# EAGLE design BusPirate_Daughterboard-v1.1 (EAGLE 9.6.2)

## Sheet 1 of 2: Power
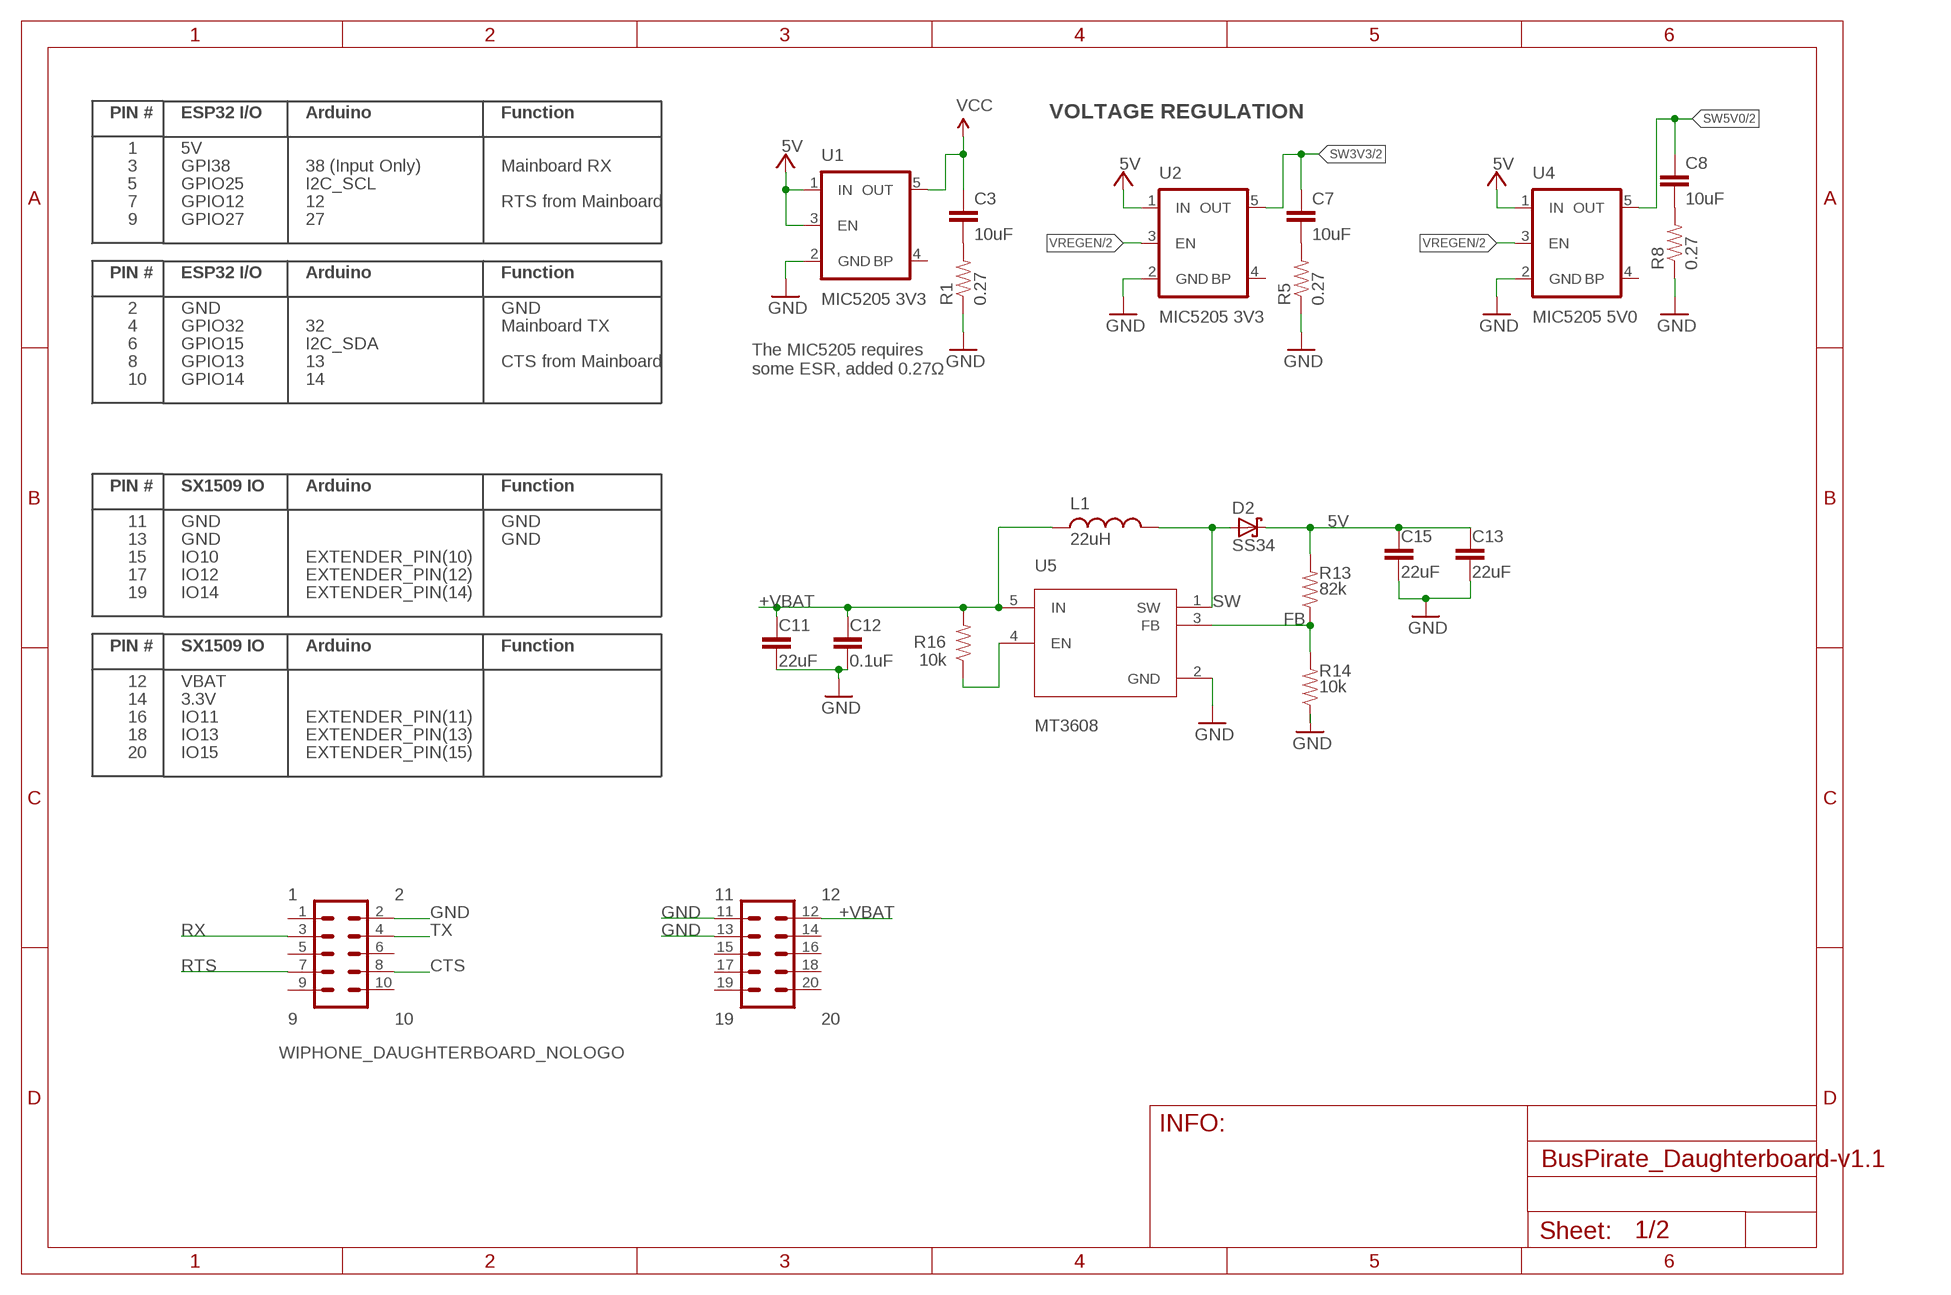
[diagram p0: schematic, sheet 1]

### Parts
C3  10uF  CAP0805  [0805_CAP]
C7  10uF  CAP0805  [0805_CAP]
C8  10uF  CAP0805  [0805_CAP]
C11  22uF  CAP0805  [0805_CAP]
C12  0.1uF  CAP0603  [0603-CAP]
C13  22uF  CAP0805  [0805_CAP]
C15  22uF  CAP0805  [0805_CAP]
D2  SS34  DIODE_SCHOTTKEY  [SOD323]
JP3  WIPHONE_DAUGHTERBOARD_NOLOGO  [WIPHONE_DAUGHTERBOARD-NL]
L1  22uH  IND0420  [0420-IND]
R1  0.27  RES0603  [0603-RES]
R5  0.27  RES0603  [0603-RES]
R8  0.27  RES0603  [0603-RES]
R13  82k  RES0603  [0603-RES]
R14  10k  RES0603  [0603-RES]
R16  10k  RES0603  [0603-RES]
U1  MIC5205 3V3  MIC5205-3.3V  [SOT23-5(SOT95P280X130-5-M)]
U2  MIC5205 3V3  MIC5205-3.3V  [SOT23-5(SOT95P280X130-5-M)]
U4  MIC5205 5V0  MIC5205-5V  [SOT23-5(SOT95P280X130-5-M)]
U5  MT3608  [SOT95P280X145-6N]

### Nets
5V: C13.2 C15.2 D2.C R13.2 U1.1(IN) U1.3(EN) U2.1(IN) U4.1(IN) ; also sheet 2
+VBAT: C11.2 C12.2 JP3.12 L1.1 R16.2 U5.5(IN)
CTS: JP3.8 ; also sheet 2
FB: R13.1 R14.2 U5.3(FB)
GND: C11.1 C12.1 C13.1 C15.1 JP3.2 JP3.11 JP3.13 R1.1 R5.1 R8.1 R14.1 U1.2(GND) U2.2(GND) U4.2(GND) U5.2(GND) ; also sheet 2
N$8: C3.2 R1.2
N$10: C7.2 R5.2
N$11: C8.2 R8.2
N$12: R16.1 U5.4(EN)
RTS: JP3.7 ; also sheet 2
RX: JP3.3 ; also sheet 2
SW: D2.A L1.2 U5.1(SW)
SW3V3: C7.1 U2.5(OUT) ; also sheet 2
SW5V0: C8.1 U4.5(OUT) ; also sheet 2
TX: JP3.4 ; also sheet 2
VCC: C3.1 U1.5(OUT) ; also sheet 2
VREGEN: U2.3(EN) U4.3(EN) ; also sheet 2
Unconnected: JP3.5 JP3.6 JP3.9 JP3.10 JP3.15 JP3.16 JP3.17 JP3.18 JP3.19 JP3.20 U1.4(BP) U2.4(BP) U4.4(BP)

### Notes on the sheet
- VOLTAGE REGULATION
- Mainboard RX
- RTS from Mainboard
- GND
- Mainboard TX
- CTS from Mainboard
- The MIC5205 requires
  some ESR, added 0.27Ω
- GND
- GND

## Sheet 2 of 2: Microcontroller
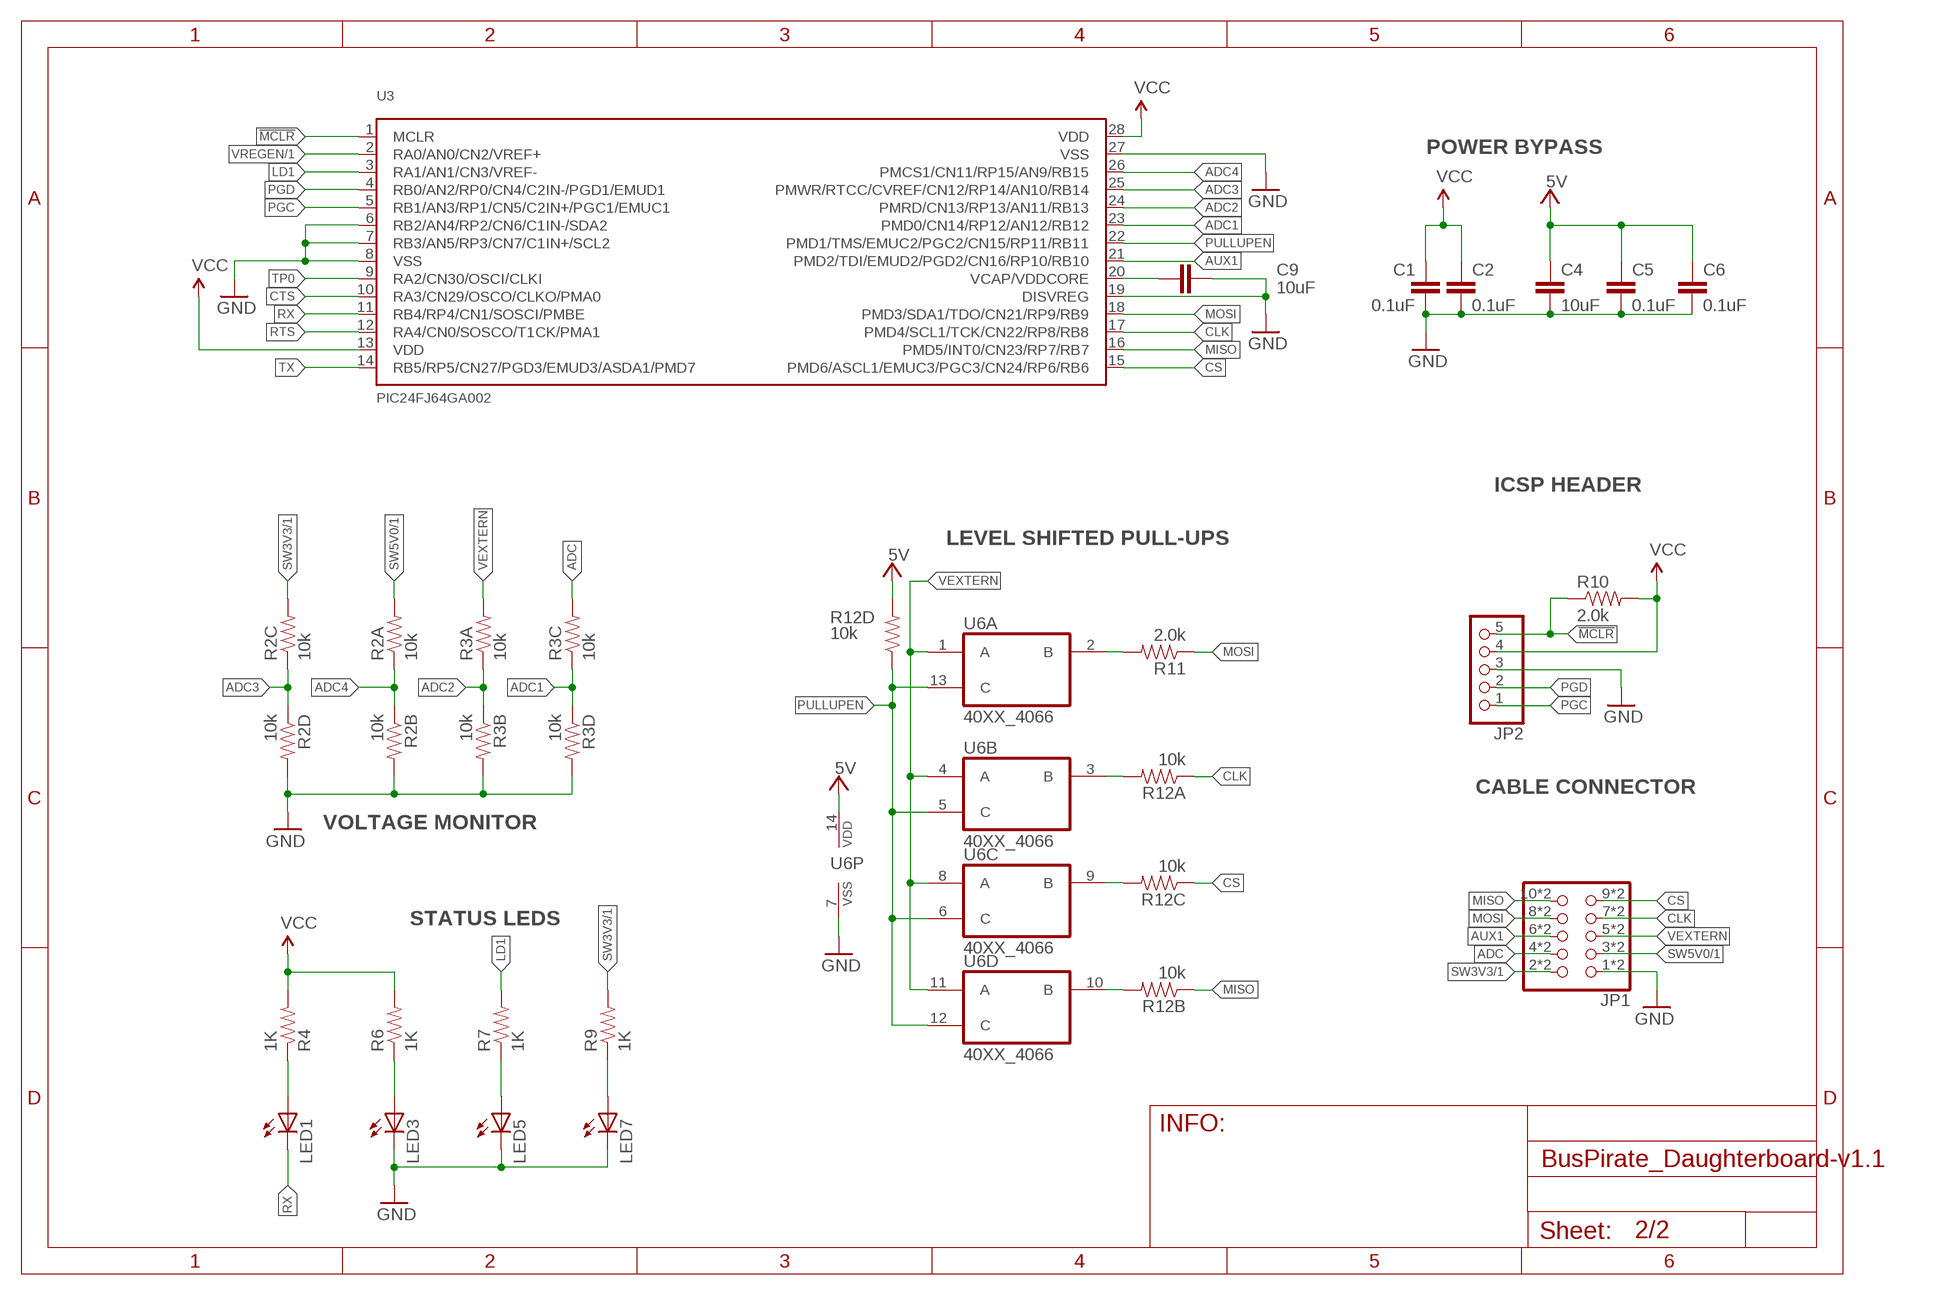
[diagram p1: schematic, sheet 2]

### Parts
C1  0.1uF  CAP0603  [0603-CAP]
C2  0.1uF  CAP0603  [0603-CAP]
C4  10uF  CAP0805  [0805_CAP]
C5  0.1uF  CAP0603  [0603-CAP]
C6  0.1uF  CAP0603  [0603-CAP]
C9  10uF  CAP0805  [0805_CAP]
JP1  PINHD-2X5-M05X2SHD_SMD  [M05X2SHD_SMD]
JP2  PINHD-1X5  [1X05]
LED1  RED  LED0603  [0603-LED]
LED3  RED  LED0603  [0603-LED]
LED5  RED  LED0603  [0603-LED]
LED7  RED  LED0603  [0603-LED]
R2  10k  RES_CAY16-F4  [RES_4XARRAY]
R3  10k  RES_CAY16-F4  [RES_4XARRAY]
R4  1K  RES0603  [0603-RES]
R6  1K  RES0603  [0603-RES]
R7  1K  RES0603  [0603-RES]
R9  1K  RES0603  [0603-RES]
R10  2.0k  RES0603  [0603-RES]
R11  2.0k  RES0603  [0603-RES]
R12  10k  RES_CAY16-F4  [RES_4XARRAY]
U3  PIC24FJ64GA002  [SSOP-28(SSOP65P780X200-28-M)]
U6  40XX_4066  [TSSOP-14(SOP65P660X120-14-M)]

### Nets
5V: C4.1 C5.1 C6.1 R12.5 U6.14(P:VDD) ; also sheet 1
!MCLR: JP2.5 R10.1 U3.1(MCLR)
ADC: JP1.4 JP1.14 R3.6
ADC1: R3.3 R3.4 U3.23(PMD0/CN14/RP12/AN12/RB12)
ADC2: R3.1 R3.2 U3.24(PMRD/CN13/RP13/AN11/RB13)
ADC3: R2.3 R2.4 U3.25(PMWR/RTCC/CVREF/CN12/RP14/AN10/RB14)
ADC4: R2.1 R2.2 U3.26(PMCS1/CN11/RP15/AN9/RB15)
AUX1: JP1.6 JP1.16 U3.21(PMD2/TDI/EMUD2/PGD2/CN16/RP10/RB10)
CLK: JP1.7 JP1.17 R12.1 U3.17(PMD4/SCL1/TCK/CN22/RP8/RB8)
CS: JP1.9 JP1.19 R12.3 U3.15(PMD6/ASCL1/EMUC3/PGC3/CN24/RP6/RB6)
CTS: U3.10(RA3/CN29/OSCO/CLKO/PMA0) ; also sheet 1
GND: C1.2 C2.2 C4.2 C5.2 C6.2 C9.2 JP1.1 JP1.11 JP2.3 LED3.C LED5.C LED7.C R2.5 R2.7 R3.5 R3.7 U3.6(RB2/AN4/RP2/CN6/C1IN-/SDA2) U3.7(RB3/AN5/RP3/CN7/C1IN+/SCL2) U3.8(VSS) U3.19(DISVREG) U3.27(VSS) U6.7(P:VSS) ; also sheet 1
LD1: R7.2 U3.3(RA1/AN1/CN3/VREF-)
MISO: JP1.10 JP1.20 R12.2 U3.16(PMD5/INT0/CN23/RP7/RB7)
MOSI: JP1.8 JP1.18 R11.1 U3.18(PMD3/SDA1/TDO/CN21/RP9/RB9)
N$1: R11.2 U6.2(A:B)
N$2: R12.6 U6.9(C:B)
N$3: C9.1 U3.20(VCAP/VDDCORE)
N$4: R12.7 U6.10(D:B)
N$5: R12.8 U6.3(B:B)
N$6: LED5.A R7.1
N$7: LED3.A R6.1
N$13: LED1.A R4.1
N$18: LED7.A R9.1
PGC: JP2.1 U3.5(RB1/AN3/RP1/CN5/C2IN+/PGC1/EMUC1)
PGD: JP2.2 U3.4(RB0/AN2/RP0/CN4/C2IN-/PGD1/EMUD1)
PULLUPEN: R12.4 U3.22(PMD1/TMS/EMUC2/PGC2/CN15/RP11/RB11) U6.5(B:C) U6.6(C:C) U6.12(D:C) U6.13(A:C)
RTS: U3.12(RA4/CN0/SOSCO/T1CK/PMA1) ; also sheet 1
RX: LED1.C U3.11(RB4/RP4/CN1/SOSCI/PMBE) ; also sheet 1
SW3V3: JP1.2 JP1.12 R2.6 R9.2 ; also sheet 1
SW5V0: JP1.3 JP1.13 R2.8 ; also sheet 1
TP0: U3.9(RA2/CN30/OSCI/CLKI)
TX: U3.14(RB5/RP5/CN27/PGD3/EMUD3/ASDA1/PMD7) ; also sheet 1
VCC: C1.1 C2.1 JP2.4 R4.2 R6.2 R10.2 U3.13(VDD) U3.28(VDD) ; also sheet 1
VEXTERN: JP1.5 JP1.15 R3.8 U6.1(A:A) U6.4(B:A) U6.8(C:A) U6.11(D:A)
VREGEN: U3.2(RA0/AN0/CN2/VREF+) ; also sheet 1

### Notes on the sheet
- POWER BYPASS
- ICSP HEADER
- LEVEL SHIFTED PULL-UPS
- CABLE CONNECTOR
- VOLTAGE MONITOR
- STATUS LEDS

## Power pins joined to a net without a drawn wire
1: JP3.1
14: JP3.14

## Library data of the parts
C1-C9 C11-C13 C15 = HackEDA V1.0:CAP: Capacitor.
D2 = HackEDA V1.0:DIODE_SCHOTTKEY: Schottky barrier diode
JP1 = HackEDA V1.0:PINHD-2X5: PIN HEADER; PROD_ID: CONN-09508
JP2 = HackEDA V1.0:PINHD-1X5: PIN HEADER
JP3 = WiPhone:WIPHONE_DAUGHTERBOARD
L1 = HackEDA V1.0:IND: Inductor.
LED1 LED3 LED5 LED7 = HackEDA V1.0:LED: LED.
R1 R4-R11 R13 R14 R16 = HackEDA V1.0:RES: Resistor.
R2 R3 R12 = HackEDA V1.0:RES_CAY16-F4: CAY16-F4; PROD_ID: RES-13167
U1 U2 U4 = HackEDA V1.0:MIC5205: MIC5205 150mA vreg 3.3V - VREG-00822 5V - VREG-00823
U3 = HackEDA V1.0:PIC24FJ64GA002: 16-bit General Purpose Flash Microcontroller
U5 = HackEDA V1.0:MT3608: High Efficiency 1.2MHz 2A Step Up Converter; DESCRIPTION: High Efficiency 1.2MHz 2A Step Up Converter; MF: Aerosemi Technology Co., Ltd; MP: MT3608; PACKAGE: Package
U6 = HackEDA V1.0:40XX_4066: Quad bilateral ANALOG SWITCH; PROD_ID: IC-13191

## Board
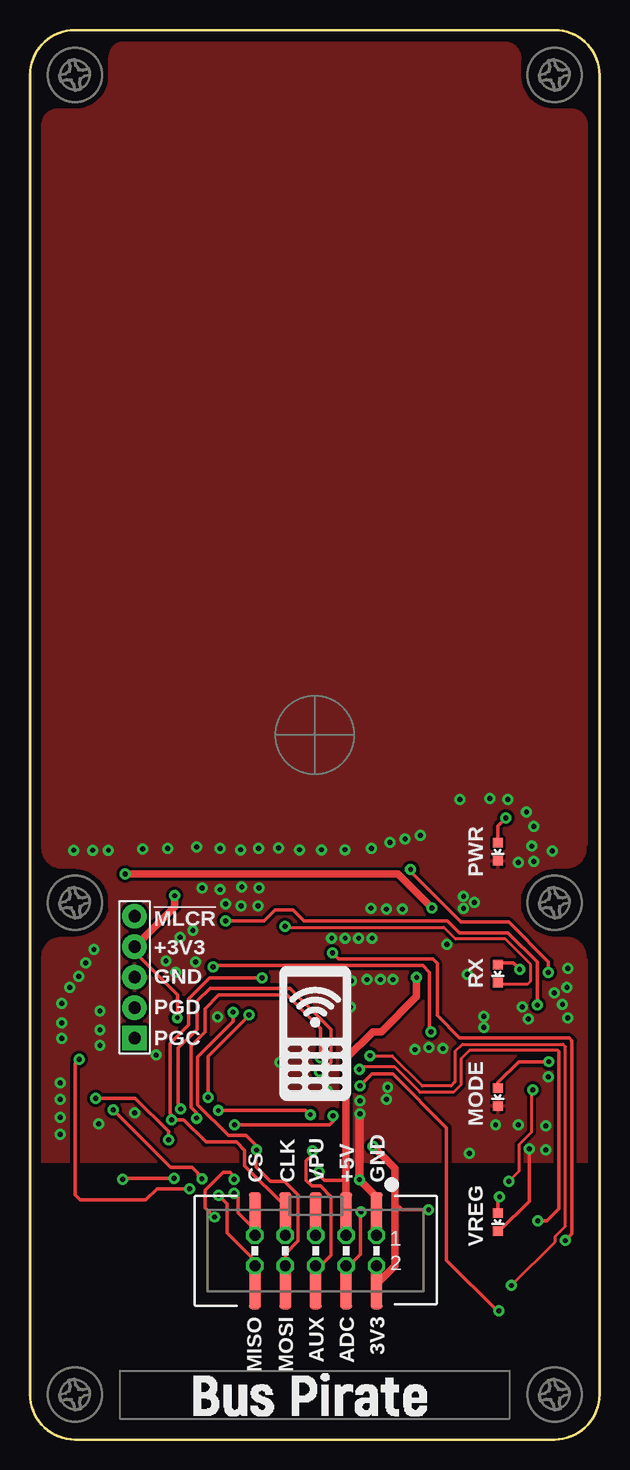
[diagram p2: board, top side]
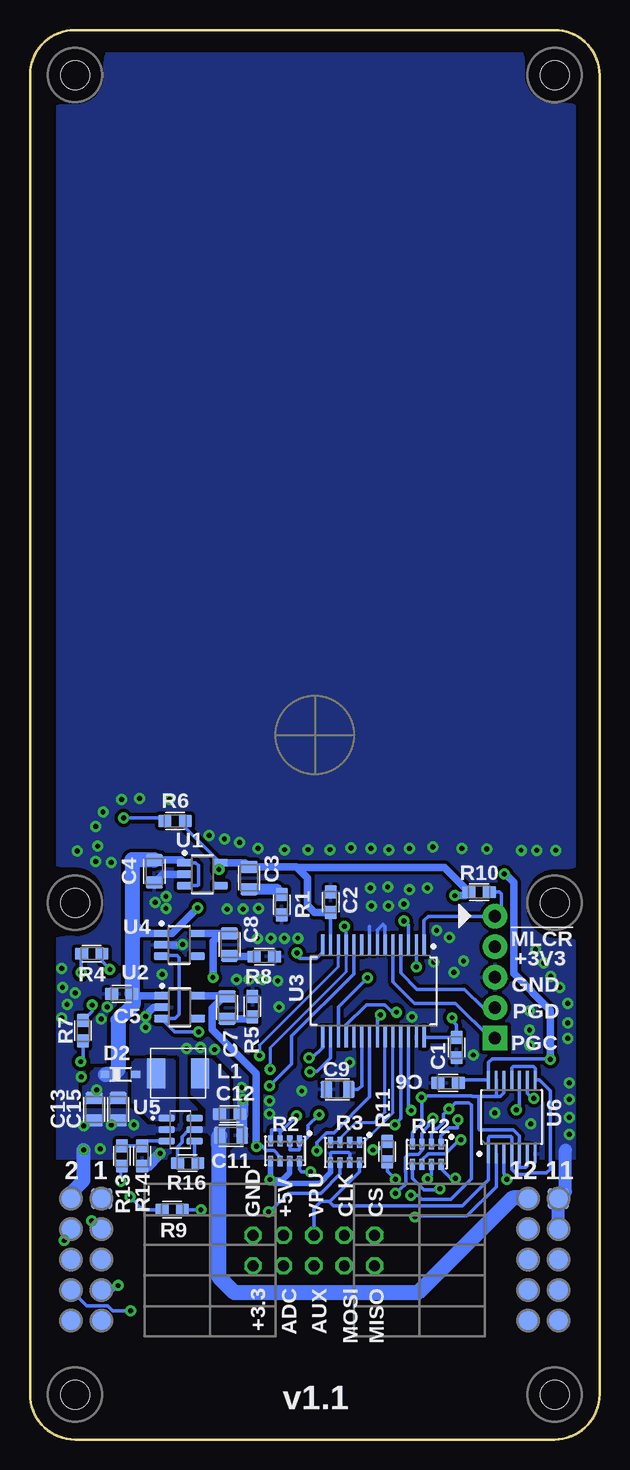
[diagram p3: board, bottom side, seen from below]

Size 47.5 x 117.5 mm. Coordinates in mm from the lower left corner, seen from the top.
Copper layers (1*16): Top 0.035mm / dielectric 1.5mm / Bottom 0.035mm
Design rules "MZJ_2Layer_Standard *": minimum track width 10mil, minimum drill 16mil, track to track 10mil, track to pad 8mil, pad to pad 8mil, via to via 10mil, smd to smd 0mil, copper to edge 8mil, drill to drill 8mil, minimum pad ring 10mil, minimum via ring 10mil, stop-mask expansion 4mil, vias tented up to drill 25mil, thermal gap 10mil
bRestrict: area 18.1,40.5 to 18.3,42.1; area 18.7,40.4 to 19,42; area 19.4,40.4 to 19.6,42; area 6.2,23 to 6.4,24.6

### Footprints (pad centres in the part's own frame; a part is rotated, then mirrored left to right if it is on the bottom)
0603-CAP = smd 1.1 x 1: 1 -0.85,0; 2 0.85,0
0805_CAP = smd 1 x 1.42: 1 -0.935,0; 2 0.935,0
SOD323 = smd 0.8 x 0.6: A 1.25,0; C -1.25,0
M05X2SHD_SMD = smd 4.15 x 1: 1 -2.794,5.08; 2 2.794,5.08; 3 -2.794,2.54; 4 2.794,2.54; 5 -2.794,0; 6 2.794,0; 7 -2.794,-2.54; 8 2.794,-2.54; 9 -2.794,-5.08; 10 2.794,-5.08 | drill 0.914 octagon: 11 -1.27,5.08; 12 1.27,5.08; 13 -1.27,2.54; 14 1.27,2.54; 15 -1.27,0; 16 1.27,0; 17 -1.27,-2.54; 18 1.27,-2.54; 19 -1.27,-5.08; 20 1.27,-5.08
1X05 = drill 1.016 pad 2.032 square: 1 -5.08,0 | drill 1.016 pad 2.032: 2 -2.54,0; 3 0,0; 4 2.54,0; 5 5.08,0
WIPHONE_DAUGHTERBOARD-NL = smd 1.75 x 1.75 bottom: 1 17.78,-38.66; 2 20.32,-38.66; 3 17.78,-41.2; 4 20.32,-41.2; 5 17.78,-43.74; 6 20.32,-43.74; 7 17.78,-46.28; 8 20.32,-46.28; 9 17.78,-48.82; 10 20.32,-48.82; 11 -20.32,-38.66; 12 -17.78,-38.66; 13 -20.32,-41.2; 14 -17.78,-41.2; 15 -20.32,-43.74; 16 -17.78,-43.74; 17 -20.32,-46.28; 18 -17.78,-46.28; 19 -20.32,-48.82; 20 -17.78,-48.82 | hole 2.4: 20,-54.991; -20,-54.991; 20,-13.991; 20,55.009; -20,55.009; -20,-13.991
0420-IND = smd 1.5 x 2.5: 1 -1.85,0; 2 1.85,0
0603-LED = smd 0.8 x 0.8: A 0,-0.75; C 0,0.75
0603-RES = smd 1.1 x 1: 1 -0.85,0; 2 0.85,0
RES_4XARRAY = smd 0.425 x 0.9: 1 -1.2,-0.85; 2 -0.4,-0.85; 3 0.4,-0.85; 4 1.2,-0.85; 5 1.2,0.85; 6 0.4,0.85; 7 -0.4,0.85; 8 -1.2,0.85
SOT23-5(SOT95P280X130-5-M) = smd 1.2 x 0.6: 1 -1.528,0.95; 2 -1.528,0; 3 -1.528,-0.95; 4 1.528,-0.95; 5 1.528,0.95
SSOP-28(SSOP65P780X200-28-M) = smd 1.748 x 0.35: 1 -3.853,4.225; 2 -3.853,3.575; 3 -3.853,2.925; 4 -3.853,2.275; 5 -3.853,1.625; 6 -3.853,0.975; 7 -3.853,0.325; 8 -3.853,-0.325; 9 -3.853,-0.975; 10 -3.853,-1.625; 11 -3.853,-2.275; 12 -3.853,-2.925; 13 -3.853,-3.575; 14 -3.853,-4.225; 15 3.853,-4.225; 16 3.853,-3.575; 17 3.853,-2.925; 18 3.853,-2.275; 19 3.853,-1.625; 20 3.853,-0.975; 21 3.853,-0.325; 22 3.853,0.325; 23 3.853,0.975; 24 3.853,1.625; 25 3.853,2.275; 26 3.853,2.925; 27 3.853,3.575; 28 3.853,4.225
SOT95P280X145-6N = smd 1.37 x 0.59: 1 -1.17,0.95; 2 -1.17,0; 3 -1.17,-0.95; 4 1.17,-0.95; 5 1.17,0; 6 1.17,0.95
TSSOP-14(SOP65P660X120-14-M) = smd 1.562 x 0.32: 1 -3.075,1.95; 2 -3.075,1.3; 3 -3.075,0.65; 4 -3.075,0; 5 -3.075,-0.65; 6 -3.075,-1.3; 7 -3.075,-1.95; 8 3.075,-1.95; 9 3.075,-1.3; 10 3.075,-0.65; 11 3.075,0; 12 3.075,0.65; 13 3.075,1.3; 14 3.075,1.95

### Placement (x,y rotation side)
C1  11.93,32.68 270 bottom
C2  22.42,44.79 90 bottom
C3  29.23,46.8 270 bottom
C4  37.13,47.37 270 bottom
C5  39.85,37.15 180 bottom
C6  12.62,29.73 180 bottom
C7  31.06,36.02 270 bottom
C8  30.86,41.26 270 bottom
C9  21.85,29.18 180 bottom
C11  30.75,25.34 180 bottom
C12  30.85,27.14 180 bottom
C13  42.15,27.54 90 bottom
C15  40.15,27.54 90 bottom
D2  39.95,30.44 0 bottom
JP1  23.83,15.74 270 top
JP2  8.72,38.54 90 top
JP3  23.75,58.74 0 top
L1  35.15,30.54 180 bottom
LED1  39.02,38.84 180 top
LED3  39.02,49 180 top
LED5  39.02,28.55 180 top
LED7  39.02,18.13 180 top
R1  26.51,44.59 90 bottom
R2  26.23,24.06 180 bottom
R3  21.23,23.93 180 bottom
R4  42.35,40.51 180 bottom
R5  28.94,36.09 270 bottom
R6  35.4,51.56 0 bottom
R7  43.07,34.08 90 bottom
R8  27.95,40.27 180 bottom
R9  35.64,19.16 0 bottom
R10  10.05,45.64 180 bottom
R11  17.71,24 270 bottom
R12  14.41,23.78 180 bottom
R13  39.85,23.64 270 bottom
R14  38.15,23.64 90 bottom
R16  34.35,23.04 180 bottom
U1  33.12,47.12 0 bottom
U2  35.02,36.04 0 bottom
U3  18.85,37.39 270 bottom
U4  35.04,41.24 0 bottom
U5  34.95,25.84 0 bottom
U6  7.32,26.89 90 bottom

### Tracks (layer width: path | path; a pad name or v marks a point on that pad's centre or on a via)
5V  (via drill 0.41)
  Top 0.254: v39.95,21.54 40.8,22.38 40.8,24.59 41.85,25.64 41.85,29.14 v41.95,29.14
  Top 0.305: v13.31,20.9 10.6,20.9 9.66,19.96 4.19,19.96 3.75,20.4 3.75,31.35 v4.1,31.7
  Top 0.61: v33.52,44.33 30.71,47.14 v7.95,47.14
  Bottom 0.254: R13.2 39.95,22.69 v39.95,21.54 | v41.95,29.14 42.15,28.94 C13.2
  Bottom 0.305: C6.1 11.54,29.96 U6.14 9.26,29.98 9.26,31.42 8.94,31.74 4.09,31.74 4.05,31.7 v4.1,31.7 | v13.31,20.9 13.31,20.83 14.65,20.83 15.61,21.78 15.61,22.55 R12.5 | U1.3 33.51,46.17 33.45,46.24 33.45,47.84 33.68,48.07 U1.1
  Bottom 0.61: 38.6,42.39 38.4,42.19 U4.1 35.66,42.19 v33.52,44.33 | U2.1 38.84,36.99 C5.1 | v4.1,31.7 4.1,35.79 7.15,38.84 7.15,46.44 7.85,47.14 v7.95,47.14 | C4.1 34.88,48.3 U1.1
  Bottom 1.27: 39,42.79 39,48.32 37.15,48.32 C4.1 | 39,42.79 C5.1 38.91,37.06 38.91,36.2 40.15,34.96 40.15,30.84 40.55,30.44 D2.C | 39,42.79 38.6,42.39
  pour Bottom (rank 2, no thermals): 39.45,28.94 39.45,30.54 39.85,30.94 42.05,30.94 42.35,30.64 43.05,29.94 43.05,27.94 42.95,28.04 39.45,28.04
!MCLR
  Bottom 0.305: U3.1 14.63,43.28 14.29,43.62 8.06,43.62 | JP2.5 8.06,43.62 | R10.1 8.37,45.64 8.2,45.48 8.2,43.76 8.06,43.62
+VBAT
  Bottom 0.305: R16.2 35.2,24.41 34.82,24.79 34.82,25.24 34.22,25.84 U5.5
  Bottom 1.27: JP3.12 5.91,20.14 7.25,20.14 15.15,12.24 30.45,12.24 31.75,13.54 31.75,25.27 C11.2
  pour Bottom (no thermals): 33.55,25.64 32.75,25.64 32.35,25.24 32.35,24.54 31.05,24.54 30.95,24.64 30.95,30.24 32.35,31.64 34,31.64 34,28.79 32.75,27.54 32.75,26.14 32.85,26.04 33.55,26.04
ADC  (via drill 0.41)
  Top 0.305: JP1.14 JP1.4 26.37,14.26 27.55,15.44 27.55,18.94 v27.6,18.99
  Bottom 0.305: R3.6 21.63,22.15 23.25,20.53 25.95,20.53 27.55,18.94 v27.6,18.99
ADC1
  Bottom 0.254: R3.3 21.63,25.11 20.32,26.42 18.76,26.42 17.88,27.3 U3.23
  Bottom 0.305: R3.3 R3.4
ADC2
  Bottom 0.254: R3.1 19.69,24.78 17.23,27.23 U3.24
  Bottom 0.305: R3.2 20.83,24.71 20.01,24.71 20.01,24.76 R3.1
ADC3  (via drill 0.41)
  Top 0.305: v17.06,26.22 24.97,26.22 25.37,26.62 25.37,26.86 v25.26,26.97
  Bottom 0.305: U3.25 16.58,26.75 17.06,26.27 v17.06,26.22 | v25.26,26.97 26.52,25.72 | 26.52,25.72 26.63,25.6 R2.3 | R2.4 27.35,24.99 27.35,25.82 26.62,25.82 26.52,25.72
ADC4  (via drill 0.41)
  Top 0.305: v15.71,27.42 22.96,27.42 23.38,27 v23.38,27.08
  Bottom 0.305: U3.26 15.93,27.63 15.72,27.42 v15.71,27.42 | v23.38,27.08 24.29,26.17 24.29,25.25 24.63,24.91 R2.1 25.03,24.18 25.07,24.14 25.8,24.14 25.8,24.88 R2.2
AUX1  (via drill 0.41)
  Top 0.305: v23.58,24.05 23.57,24.04 23.57,23.75 23.04,23.21 23.04,21.6 23.5,21.13 24.23,21.13 25.12,20.24 25.12,15.34 23.83,14.05 JP1.6 JP1.16
  Bottom 0.305: U3.21 19.18,28.55 22.14,25.58 22.79,25.58 23.58,24.79 v23.58,24.05
CLK  (via drill 0.41)
  Top 0.305: JP1.17 JP1.7 21.29,19.42 17.89,22.82 17.89,24.12 17.21,24.8 14.67,24.8 12.83,26.64 v11.83,26.64 11.83,27.07 11.71,27.19 11.71,33.04 13.25,34.58 13.25,36.74 14.99,38.48 v19.36,38.48
  Bottom 0.305: v11.83,26.64 11.83,26.42 11.87,26.38 11.87,25.97 12.58,25.97 13.21,25.33 R12.1 | U3.17 21.78,36.07 v19.36,38.48
CS  (via drill 0.41)
  Top 0.305: v13.9,26.79 13.9,27.22 13.44,27.68 13.44,32.81 14.59,33.96 14.59,35.92 15.74,37.06 21.44,37.06 24.23,34.28 v24.23,31.8 | JP1.9 JP1.19 18.75,17.5 17.33,18.91 17.33,20.22 v17.03,20.52
  Bottom 0.305: U3.15 23.08,32.68 23.96,31.8 v24.23,31.8 | v13.9,26.79 v13.91,26.8 13.91,26.81 14.27,26.44 14.27,26.15 14.67,25.75 14.67,25.65 14.81,25.51 R12.3 14.81,24.08 15.1,23.79 15.91,23.79 16.18,23.53 16.18,22.33 16.17,22.32 16.17,21.33 16.67,20.83 16.72,20.83 v17.03,20.52
CTS  (via drill 0.41)
  Top 0.305: v27.52,29.47 28.52,30.47 30.26,30.47 34.75,25.98 34.75,14.93 38.96,10.72 v39.09,10.72
  Bottom 0.305: U3.10 20.48,38.83 25.68,33.63 25.68,31.31 v27.52,29.47 | v39.09,10.72 40.59,10.72 41.02,11.15 42.76,11.15 JP3.8
FB
  Bottom 0.305: R13.1 R14.2 37.75,24.89 U5.3
GND  (via drill 0.41)
  Top 0.305: JP1.1 JP1.11 | v41.63,24.24 41.63,19.86 39.16,17.38 LED7.C
  Top 0.61: v27.47,21.67 28.91,20.22 JP1.1
  Top 0.711: v27.47,21.67 27.47,27.08 v27.53,27.14
  Bottom 0.305: U3.6 17.88,42.76 18.06,42.94 18.53,42.47 U3.7 | U3.8 19.18,42.78 | R3.7 20.83,23.82 20.95,23.94 22.35,23.94 22.43,23.85 R3.5
  Bottom 0.457: R2.7 25.83,22.25 26.42,21.67 v27.47,21.67 | R2.5 27.43,21.7 v27.47,21.67 | R3.5 22.43,22.25 23.32,21.36 27.16,21.36 v27.47,21.67
  Bottom 0.61: v37.86,35.26 37.65,35.47 37.65,35.56 37.17,36.04 U2.2 | U4.2 34.79,41.24 v34.76,41.26 | U1.2 36.44,47.12 C4.2
  Bottom 0.914: R14.1 37.69,22.79 v36.63,23.84 | C11.1 29.81,26.95 C12.1 29.73,27.4 v29.73,28.34
  Bottom 1.067: JP3.13 JP3.11 2.85,20.66 2.85,24.14
  Bottom 1.168: JP3.2 44.07,20.58 43.03,21.62 v43.03,24.14
  other vias: 17.66,46.06 12.53,41.84 5.73,26.33 2.53,28.34 2.53,25.44 2.53,29.74 4.63,39.74 2.53,26.84 8.73,27.24 10.53,32.04 12.13,38.94 20.83,31.44 24.83,29.04 43.23,30.24 26.83,38.24 26.73,36.04 11.46,49.26 15.86,49.26 19.06,49.26 22.46,49.16 26.26,49.16 28.46,49.26 32.56,50.36 29.83,29.34 27.53,28.24 15.63,35.24 41.86,49.46 43.56,49.06 36.16,44.26 36.16,45.26 37.06,44.76 37.86,34.36 36.46,38.76 38.83,26.24 40.73,26.24 43.03,26.14 41.06,36.06 41.56,35.06 5.83,35.74 5.83,34.14 5.83,32.84 2.63,36.34 2.63,34.74 2.63,33.44 3.64,49.12 5.24,49.12 6.54,49.12 34.44,32.59 33.27,32.67 32.1,32.5 15.86,45.84 14.36,45.99 19.09,45.99 19.01,44.49 17.59,44.49 16.31,44.64 26.29,41.79 27.41,41.79 28.54,41.79 25.16,41.79 28.09,38.34 29.21,38.34 30.26,38.34 13.58,42.44 13.81,39.82 11.33,39.89 43.74,37.24 44.41,36.26 44.86,35.14 44.79,37.69 44.86,39.26 28.44,44.29 29.71,44.21 31.06,44.21 40.74,48.11 42.01,48.19 35.86,53.36 38.34,53.44 39.84,53.36 41.41,52.31 42.01,51.11 13.89,49.39 9.39,49.24 17.56,49.16 20.71,49.31 24.31,49.16 30.01,49.76 31.29,50.06 3.31,37.69 4.06,38.59 5.33,40.84
  pour Top (isolate 0.203, rank 2): 47.55,117.59 47.55,23.18 -0.04,23.18 -0.04,117.59
  pour Bottom (isolate 0.305, rank 3): 47.54,117.59 47.53,23.48 -0.04,23.48 -0.03,117.59
  pour Bottom (no thermals): 35.95,26.04 37.55,26.04 39.05,27.54 43.05,27.54 43.15,27.44 43.15,25.84 42.95,25.64 35.95,25.64
LD1  (via drill 0.41)
  Top 0.305: v16.31,43.23 19.54,43.23 20.45,44.14 21.95,44.14 22.85,43.23 34.83,43.23 35.82,42.24 39.87,42.24 42.3,39.81 v42.3,36.21
  Bottom 0.305: U3.3 15.93,42.88 16.06,43.01 16.19,43.01 16.31,43.13 v16.31,43.23 | R7.2 42.3,35.7 v42.3,36.21
MISO  (via drill 0.41)
  Top 0.305: v24.14,30.63 24.45,30.94 24.59,30.94 25.09,31.44 25.09,34.2 21.68,37.62 15,37.62 13.93,36.55 13.93,34.2 12.37,32.65 12.37,27.74 v12.57,27.55 | JP1.10 JP1.20 18.75,14.9 16.43,17.22 16.43,19.65 v15.73,20.34
  Bottom 0.305: U3.16 22.43,31.82 23.57,30.68 23.91,30.68 23.96,30.63 v24.14,30.63 | R12.2 14.01,25.51 13.6,25.92 13.54,25.92 13.03,26.43 13.03,27.08 v12.57,27.55 12.04,28.08 10.88,28.08 10.7,27.9 10.7,21.73 12.39,20.04 14.83,20.04 15.14,20.34 v15.73,20.34
MOSI  (via drill 0.41)
  Top 0.305: v16.95,35.62 16.95,34.84 13.99,31.88 13.99,27.91 16.55,25.35 18.01,25.35 18.91,24.46 v18.91,24.13 18.86,24.08 18.86,22.71 20.05,21.52 21.23,21.52 22.36,20.4 22.36,16.56 21.29,15.5 JP1.18 JP1.8
  Bottom 0.305: U3.18 21.13,34.55 19.43,36.24 17.92,36.24 17.31,35.64 v16.97,35.64 v16.95,35.62 | R11.1 18.43,24.13 v18.91,24.13
N$1  (via drill 0.41)
  Top 0.305: v15.39,18.54 14.62,19.32 14.62,20.79 16.11,22.29 16.67,22.29 17.16,21.8 17.16,21.63 17.09,21.63 v17.03,21.69
  Bottom 0.305: U6.2 8.62,21.07 11.05,18.64 15.29,18.64 v15.39,18.54 | v17.03,21.69 17.71,22.37 R11.2
N$2  (via drill 0.41)
  Top 0.305: v11.57,24.97 11.57,25.67 8.79,28.45 5.69,28.45 5.68,28.43 v5.48,28.43
  Bottom 0.305: v11.57,24.97 11.72,24.81 11.86,24.81 12.85,23.82 14.28,23.82 14.81,23.29 R12.6 | U6.9 6.02,28.83 5.62,28.43 v5.48,28.43
N$3
  Bottom 0.305: C9.1 20.13,29.18 19.83,29.49 U3.20
N$4  (via drill 0.41)
  Top 0.305: v6.93,27.49 11.75,22.68 13.53,22.68 14.03,22.18 14.03,22.04 v14.34,21.73
  Bottom 0.305: U6.10 6.67,27.74 6.92,27.49 v6.93,27.49 | R12.7 14.01,22.2 14.03,22.18 14.03,22.04 v14.34,21.73
N$5  (via drill 0.41)
  Top 0.305: v12.03,21.77 7.81,21.77 v7.72,21.68
  Bottom 0.305: U6.3 7.97,22.2 7.76,21.98 7.76,21.72 v7.72,21.68 | R12.8 13.21,22.58 12.39,21.77 v12.03,21.77
N$6  (via drill 0.41)
  Top 0.305: v43.26,31.5 40.76,31.5 39.02,29.76 LED5.A
  Bottom 0.305: v43.26,31.5 43.07,31.69 R7.1
N$7  (via drill 0.41)
  Top 0.305: v39.69,51.82 39.69,51.79 39.02,51.13 LED3.A
  Bottom 0.305: R6.1 36.5,51.82 v39.69,51.82
N$8
  Bottom 0.914: R1.2 26.94,45.86 C3.2
N$10
  Bottom 0.61: R5.2 29.12,35.07 29.13,35.08 C7.2
N$11
  Bottom 0.61: R8.2 30.8,40.27 C8.2
N$12
  Bottom 0.305: U5.4 33.78,23.32 R16.1
N$13  (via drill 0.41)
  Top 0.305: v40.84,39.18 40.29,39.72 39.16,39.72 LED1.A
  Bottom 0.305: R4.1 41.5,39.84 v40.84,39.18
N$18  (via drill 0.41)
  Top 0.305: LED7.A 39.02,20.09 v39.17,20.24
  Bottom 0.305: R9.1 38.09,19.16 v39.17,20.24
PGC
  Bottom 0.305: JP2.1 9.1,33.46 12.01,36.37 15.44,36.37 17.23,38.16 U3.5
PGD
  Bottom 0.305: JP2.2 9.75,36 11.29,37.54 15.24,37.54 16.58,38.88 U3.4
PULLUPEN  (via drill 0.41)
  Top 0.305: v18.27,35.38 v18.27,35.37 14.86,31.95 v14.86,28.52
  Bottom 0.305: U3.22 18.53,35.13 v18.27,35.38 | R12.4 15.61,25.6 14.83,26.38 14.83,28.55 | U6.12 7.97,28.89 8.27,28.6 8.7,28.6 | 8.7,28.6 10.07,28.6 | 10.07,28.6 10.61,28.6 10.65,28.64 14.74,28.64 14.83,28.55 | U6.13 8.62,28.67 8.7,28.6 | 10.07,28.6 10.07,25.89 10.01,25.83 7.2,25.83 6.67,25.31 U6.5 6.67,22.67 6.16,22.67 6.02,22.8 U6.6 | 14.83,28.55 v14.86,28.52
RTS  (via drill 0.41)
  Top 0.254: v28.37,32 30.2,32 32.73,29.48 35.13,29.48 35.46,29.81 35.46,32.34 36.06,32.94 44.45,32.94 44.66,32.74 44.66,17.78 43.81,16.93 43.81,16.5 v40.15,12.84
  Bottom 0.254: U3.12 21.78,39.46 28.37,32.87 v28.37,32
  Bottom 0.305: JP3.7 40.52,12.46 v40.15,12.84
RX  (via drill 0.41)
  Top 0.254: v27.46,30.86 27.66,31.06 30.43,31.06 32.52,28.97 35.34,28.97 35.96,29.6 35.96,31.75 36.65,32.44 44.05,32.44 44.12,32.37 | v21.27,42.77 21.43,42.77 21.51,42.7 34.52,42.7 35.5,41.71 39.65,41.71 41.77,39.59 41.77,38.24 41.48,37.95 39.16,37.95 LED1.C
  Top 0.305: v42.35,18.24 43.12,18.24 44.12,19.24 44.12,32.37
  Bottom 0.254: U3.11 21.13,38.99 27.46,32.65 v27.46,30.86
  Bottom 0.305: JP3.3 41.65,17.54 v42.35,18.24 | U3.11 21.13,42.63 v21.27,42.77
SW
  pour Bottom (no thermals): 35.45,26.74 35.45,31.54 35.55,31.64 38.75,31.64 38.95,31.44 38.95,28.14 37.45,26.64 35.55,26.64
SW3V3  (via drill 0.41)
  Top 0.305: JP1.2 28.91,14.44 JP1.12 | v33.25,19.14 31.05,19.14 30.45,19.74
  Top 0.61: v28.6,24.44 30.45,22.59 30.45,19.74 30.45,14.48 JP1.2 | 28.91,12.29 28.91,14.44
  Bottom 0.305: R2.6 26.63,23.57 27.16,24.1 27.79,24.1 28.16,24.46 28.63,24.46 | R9.2 33.27,19.16 v33.25,19.14
  Bottom 0.61: v28.6,24.44 28.63,24.46 28.63,30.52 32.32,34.21 32.32,35.93 31.29,36.95 C7.1 31.1,36.99 U2.5
SW5V0  (via drill 0.41)
  Top 0.305: 26.37,21.6 24.56,21.6 24.11,22.05 v24.11,22.3 | JP1.3 JP1.13
  Top 0.61: JP1.3 26.37,21.6 26.37,31.76 28.61,34 29.31,34 | 29.31,34 29.32,34 | 29.31,34 32.25,36.93 v32.25,38.54
  Bottom 0.305: v24.11,22.3 24.14,22.33 24.85,22.33 25.03,22.51 R2.8
  Bottom 0.61: v32.25,38.54 32.25,41.54 31.6,42.19 | U4.5 31.6,42.19 | C8.1 31.6,42.19
TX  (via drill 0.41)
  Top 0.305: v25.23,40.56 25.73,40.07 33.59,40.07 33.97,39.69 33.97,35.33 35.83,33.48 44.96,33.48 45.2,33.24 45.2,17.14 v44.65,16.59
  Bottom 0.305: U3.14 23.08,40.65 23.61,40.12 25.03,40.12 25.23,40.32 v25.23,40.56 | JP3.4 44.65,16.96 v44.65,16.59
VCC  (via drill 0.41)
  Top 0.305: v12.29,35.17 12.29,37.07 8.72,40.64 JP2.4 | v43.24,38.93 43.24,39.83 39.92,43.15 35.94,43.15 31.75,47.34 v31.75,47.54
  Top 0.61: JP2.4 12.05,44.41 v12.05,45.34
  Bottom 0.305: U3.13 22.43,43.93 C2.1 | U3.28 11.94,33.54 C1.1 11.93,34.56 12.25,34.89 12.25,35.13 v12.29,35.17 | R6.2 34.55,51.02 U1.5 31.59,47.69 v31.75,47.54 | R4.2 43.24,40.47 v43.24,38.93
  Bottom 0.61: 25.25,47.7 12.95,47.7 R10.2 11.2,45.34 v12.05,45.34 | C2.1 23.75,43.94 24.35,44.54 24.35,46.8 25.25,47.7 | 25.25,47.7 25.28,47.73 C3.1 29.57,48.07 U1.5
VEXTERN
  Top 0.305: 23.83,19.46 JP1.5 JP1.15
  Bottom 0.305: R3.8 20.03,22.3 22.49,19.84 22.55,19.84 | U6.11 7.32,30.96 7.19,31.1 5.52,31.1 5.37,30.95 U6.8 5.03,29.96 4.11,29.04 4.11,22.53 4.42,22.22 5.81,22.22 5.93,22.11 6.91,22.11 7.32,22.53 U6.4 7.32,25.17 7.42,25.26 9.17,25.26 9.27,25.15 U6.1 9.27,21.65 11.44,19.48 22.19,19.48 22.55,19.84 | 22.55,19.84 23.25,19.84 23.83,19.25 JP1.15
VREGEN  (via drill 0.41)
  Top 0.305: v15.26,39.41 15.26,39.43 15.42,39.58 15.49,39.51 32.76,39.51 33.32,38.95 33.32,34.1 v33.44,33.98
  Bottom 0.305: U3.2 15.28,39.42 v15.26,39.41 | v33.44,33.98 35.43,33.98 U2.3 35.39,35.09 35.05,35.44 35.05,40.14 35.25,40.34 36.52,40.34 U4.3

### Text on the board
tPlace: PWR | !MLCR | +3V3 | GND | RX | PGD | PGC | MODE | CS | CLK | VPU | +5V | GND | VREG | MISO | MOSI | AUX | ADC | 3V3
bPlace: !MLCR | +3V3 | GND | PGD | PGC | v1.1
bNames: CS | CLK | VPU | +5V | GND | MISO | MOSI | AUX | ADC | +3.3
Reference: Programming Header | I/O header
